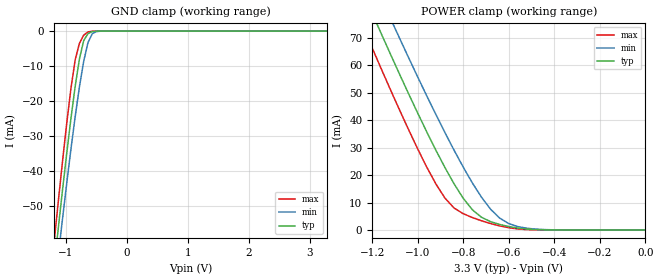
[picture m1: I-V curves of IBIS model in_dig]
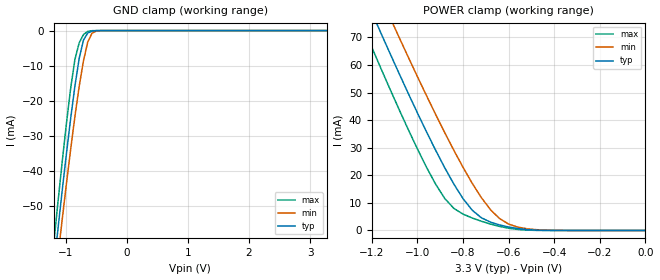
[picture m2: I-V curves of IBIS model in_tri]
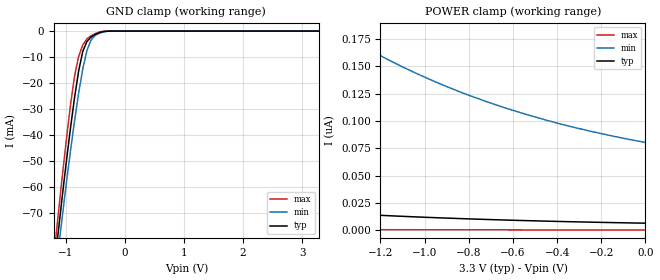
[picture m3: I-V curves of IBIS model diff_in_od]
| Integrated Devices Technolgy, Inc
[Ibis Ver]   4.1
[File Name]   9zml1252e.ibs
[File Rev]   1.1
[Date]   Friday, November 3, 2017
[Source]   Integrated Devices Technolgy, Inc.
[Notes]   Rev 1.1 created by EvK
|   Rev 1.0 to 1.1: Updated LP-HCSL output model
[Disclaimer] Integrated Device Technology, Inc. ("IDT") hereby grants the
   user of this IBIS model a non-exclusive, nontransferable
   license to use this IBIS model under the following terms. The
   user is granted this license only to use the IBIS model and is
   not granted rights to sell, copy (except as needed to run the
   IBIS model), rent, lease or sub-license the IBIS model in
   whole or in part, or in modified form to anyone. The User may
   modify the IBIS model to suit its specific applications, but
   rights to derivative works and such modifications shall belong
   to IDT. This IBIS model is provided on an AS IS" basis and IDT
   makes absolutely no warranty with respect to the information
   contained herein. IDT DISCLAIMS AND CUSTOMER WAIVES ALL
   WARRANTIES, EXPRESS AND IMPLIED, INCLUDING WARRANTIES OF
   MERCHANTABILITY AND FITNESS FOR A PARTICULAR PURPOSE. THE
   ENTIRE RISK AS TO QUALITY AND PERFORMANCE IS WITH THE USER
   ACCORDINGLY, IN NO EVENT SHALL IDT BE LIABLE FOR ANY DIRECT OR
   INDIRECT DAMAGES, WHETHER IN CONTRACT OR TORT, INCLUDING ANY
   LOST PROFITS OR OTHER INCIDENTAL, CONSEQUENTIAL, EXEMPLARY, OR
   PUNITIVE DAMAGES ARISING OUT OF THE USE OR APPLICATION OF THE
   IBIS model. Further, IDT reserves the right to make changes
   without notice to any product herein to improve reliability,
   function, or design. IDT does not convey any license under
   patent rights or any other intellectual property rights,
   including those of third parties. IDT is not obligated to
   provide maintenance or support for the licensed IBIS model.
   (C) Copyright Integrated Device Technology, Inc. 2016 All
   rights reserved
|   COMPONENT: 9ZML1252E
[Component]   9ZML1252E
[Manufacturer]   Integrated Device Technology, Inc.
[Package]
| variable   typ   min   max
R_pkg   81.10m   62.20m   100.00m
L_pkg   6.70nH   4.90nH   8.50nH
C_pkg   0.53pF   0.21pF   0.85pF
[Pin]   signal_name   model_name   R_pin   L_pin   C_pin
1   VDDA   POWER
2   GNDA   GND
3   SEL_A_B#   in_dig
4   HBW_BYP_LOBW#  in_tri
5   CKPWRGD#   in_dig
6   DIF_INB   diff_in_od
7   DIF_INB#   diff_in_od
8   GND   GND
9   VDDR   POWER
10   DIF_INA   diff_in_od
11   DIF_INA#   diff_in_od
12   SADR0_TRI   in_tri_od
13   SMBDAT   sda_od
14   SMBCLK   scl_od
15   SADR1_TRI   in_tri_od
16   NC   NC
17   FBOUT_NC#   NC
18   FBOUT_NC   NC
19   OE_0#   in_dig
20   OE_1#   in_dig
21   NC   NC
22   GND   GND
23   DIF_0   diff_out
24   DIF_0#   diff_out
25   DIF_1   diff_out
26   DIF_1#   diff_out
27   GND   GND
28   VDD   POWER
29   DIF_2   diff_out
30   DIF_2#   diff_out
31   DIF_3   diff_out
32   DIF_3#   diff_out
33   NC   NC
34   GND   GND
35   OE_2#   in_dig
36   OE_3#   in_dig
37   OE_4#   in_dig
38   OE_5#   in_dig
39   GND   GND
40   VDDIO   POWER
41   DIF_4   diff_out
42   DIF_4#   diff_out
43   DIF_5   diff_out
44   DIF_5#   diff_out
45   VDD   POWER
46   GND   GND
47   DIF_6   diff_out
48   DIF_6#   diff_out
49   DIF_7   diff_out
50   DIF_7#   diff_out
51   GND   GND
52   VDDIO   POWER
53   OE_6#   in_dig
54   OE_7#   in_dig
55   OE_8#   in_dig
56   OE_9#   in_dig
57   NC   NC
58   GND   GND
59   DIF_8   diff_out
60   DIF_8#   diff_out
61   DIF_9   diff_out
62   DIF_9#   diff_out
63   GND   GND
64   VDD   POWER
65   DIF_10   diff_out
66   DIF_10#   diff_out
67   DIF_11   diff_out
68   DIF_11#   diff_out
69   NC   NC
70   GND   GND
71   OE_10#   in_dig
72   OE_11#   in_dig
73   EPAD   GND
[Diff Pin]   inv_pin   vdiff   tdelay_typ
6   7   NA   NA
10   11   NA   NA
23   24   NA   NA
25   26   NA   NA
29   30   NA   NA
31   32   NA   NA
41   42   NA   NA
43   44   NA   NA
47   48   NA   NA
49   50   NA   NA
59   60   NA   NA
61   62   NA   NA
65   66   NA   NA
67   68   NA   NA
| Models and submodels in the file (7): in_dig (Input), in_tri (Input), diff_in_od (Input), in_tri_od (Input), sda_od (I/O_open_drain), scl_od (Input), diff_out (Output)
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|   Model in_dig
[Model]  in_dig
Model_type Input
Polarity   Non-Inverting
Vinl =   0.8000V
Vinh =   2.0000V
C_comp   2.1000pF   2.1000pF   2.1000pF
[Temperature Range]   25.0000   85.0000   -40.0000
[Voltage Range]   3.3000V   3.1350V   3.4650V
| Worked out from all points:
|   GND clamp passes 1 mA (typ) near -0.65 V on its own axis
|   POWER clamp passes 1 mA (typ) near -0.58 V on its own axis
[GND_clamp]
|Voltage   I(typ)   I(min)   I(max)
-3.3V     -444.4mA   -436.3mA   -455.2mA
-1.2V     -68.37mA   -75.7mA    -61.37mA
-1.13V    -56.99mA   -64.8mA    -49.35mA
-1.06V    -45.92mA   -54.16mA   -37.72mA
-920mV    -25.14mA   -33.91mA   -16.51mA
-850mV    -15.84mA   -24.53mA   -8.255mA
-780mV    -7.95mA    -15.96mA   -3.499mA
-710mV    -2.728mA   -8.626mA   -1.156mA
-640mV    -697.7uA   -3.286mA   -240.6uA
-570mV    -146.6uA   -751uA     -34.01uA
-430mV    -3.844uA   -23.08uA   -279.3nA
3.28V     213.4pA    44.16nA    205.9pA
[POWER_clamp]
|Voltage   I(typ)   I(min)   I(max)
-3.28V    509.3mA    515.8mA    504.9mA
-1.24V    86.61mA    99.33mA    74.1mA
-1.16V    71.55mA    84.5mA     58.72mA
-1.12V    64.14mA    77.19mA    51.18mA
-1.08V    56.84mA    69.96mA    43.78mA
-960mV    35.71mA    48.84mA    22.88mA
-880mV    22.69mA    35.43mA    11.57mA
-840mV    16.77mA    29.02mA    7.979mA
-760mV    7.367mA    17.14mA    4.53mA
-640mV    2.005mA    4.321mA    1.477mA
-480mV    131.2uA    293.3uA    37.64uA
0V        220.8pA    394.5pA    228.5pA
|   Model in_tri
[Model]  in_tri
Model_type Input
Polarity   Non-Inverting
Vinl =   0.8000V
Vinh =   2.0000V
C_comp   2.1400pF   2.1400pF   2.1400pF
[Temperature Range]   25.0000   85.0000   -40.0000
[Voltage Range]   3.3000V   3.1350V   3.4650V
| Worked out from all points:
|   GND clamp passes 1 mA (typ) near -0.65 V on its own axis
|   POWER clamp passes 1 mA (typ) near -0.58 V on its own axis
[GND_clamp]
|Voltage   I(typ)   I(min)   I(max)
-3.3V     -444.4mA   -436.3mA   -455.2mA
-1.2V     -68.37mA   -75.7mA    -61.37mA
-1.13V    -56.99mA   -64.8mA    -49.35mA
-1.06V    -45.92mA   -54.16mA   -37.72mA
-920mV    -25.14mA   -33.91mA   -16.51mA
-850mV    -15.84mA   -24.53mA   -8.255mA
-780mV    -7.95mA    -15.96mA   -3.499mA
-710mV    -2.728mA   -8.625mA   -1.156mA
-640mV    -697.7uA   -3.286mA   -240.6uA
-570mV    -146.6uA   -751uA     -34.01uA
-430mV    -3.844uA   -23.08uA   -279.3nA
3.28V     213.4pA    44.16nA    205.9pA
[POWER_clamp]
|Voltage   I(typ)   I(min)   I(max)
-3.28V    509.3mA    515.8mA    504.9mA
-1.24V    86.61mA    99.33mA    74.1mA
-1.16V    71.55mA    84.5mA     58.72mA
-1.12V    64.14mA    77.19mA    51.18mA
-1.08V    56.84mA    69.96mA    43.78mA
-960mV    35.71mA    48.84mA    22.88mA
-880mV    22.69mA    35.43mA    11.57mA
-840mV    16.77mA    29.02mA    7.979mA
-760mV    7.367mA    17.14mA    4.53mA
-640mV    2.005mA    4.321mA    1.477mA
-480mV    131.2uA    293.3uA    37.64uA
0V        220.8pA    394.5pA    228.4pA
|   Model diff_in_od
[Model]  diff_in_od
Model_type Input
Polarity   Non-Inverting
Vinl =   0.3000V
Vinh =   0.5000V
C_comp   3.5000pF   3.5000pF   3.5000pF
[Temperature Range]   25.0000   85.0000   -40.0000
[Voltage Range]   3.3000V   3.1350V   3.4650V
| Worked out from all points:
|   GND clamp passes 1 mA (typ) near -0.47 V on its own axis
[GND_clamp]
|Voltage   I(typ)   I(min)   I(max)
-3.3V     -581.4mA   -566.8mA   -600.3mA
-1.2V     -92.9mA    -99.3mA    -87.17mA
-1.13V    -78.34mA   -85.45mA   -71.6mA
-1.06V    -64.19mA   -71.96mA   -56.52mA
-920mV    -37.64mA   -46.39mA   -28.76mA
-850mV    -25.69mA   -34.6mA    -17.37mA
-780mV    -15.32mA   -23.82mA   -9.726mA
-710mV    -7.779mA   -14.52mA   -5.31mA
-640mV    -3.984mA   -7.427mA   -3.004mA
-500mV    -1.282mA   -1.675mA   -939.5uA
-220mV    -3.662uA   -14.35uA   -357.2nA
3.28V     6.54nA     86.14nA    391.5pA
[POWER_clamp]
|Voltage   I(typ)   I(min)   I(max)
-3.28V    57.48nA    654.6nA    1.522nA
-2.84V    43.19nA    492.3nA    1.256nA
-2.4V     32.05nA    365.8nA    1.04nA
-1.92V    22.9nA     262.2nA    852pA
-1.4V     15.85nA    182.8nA    693.7pA
-1.12V    13.05nA    151.5nA    623.8pA
-960mV    11.71nA    136.6nA    587.9pA
-800mV    10.54nA    123.6nA    554.6pA
-640mV    9.52nA     112.3nA    523.5pA
-440mV    8.427nA    100.3nA    487.7pA
-240mV    7.511nA    90.3nA     454.6pA
0V        6.607nA    80.43nA    417.9pA
